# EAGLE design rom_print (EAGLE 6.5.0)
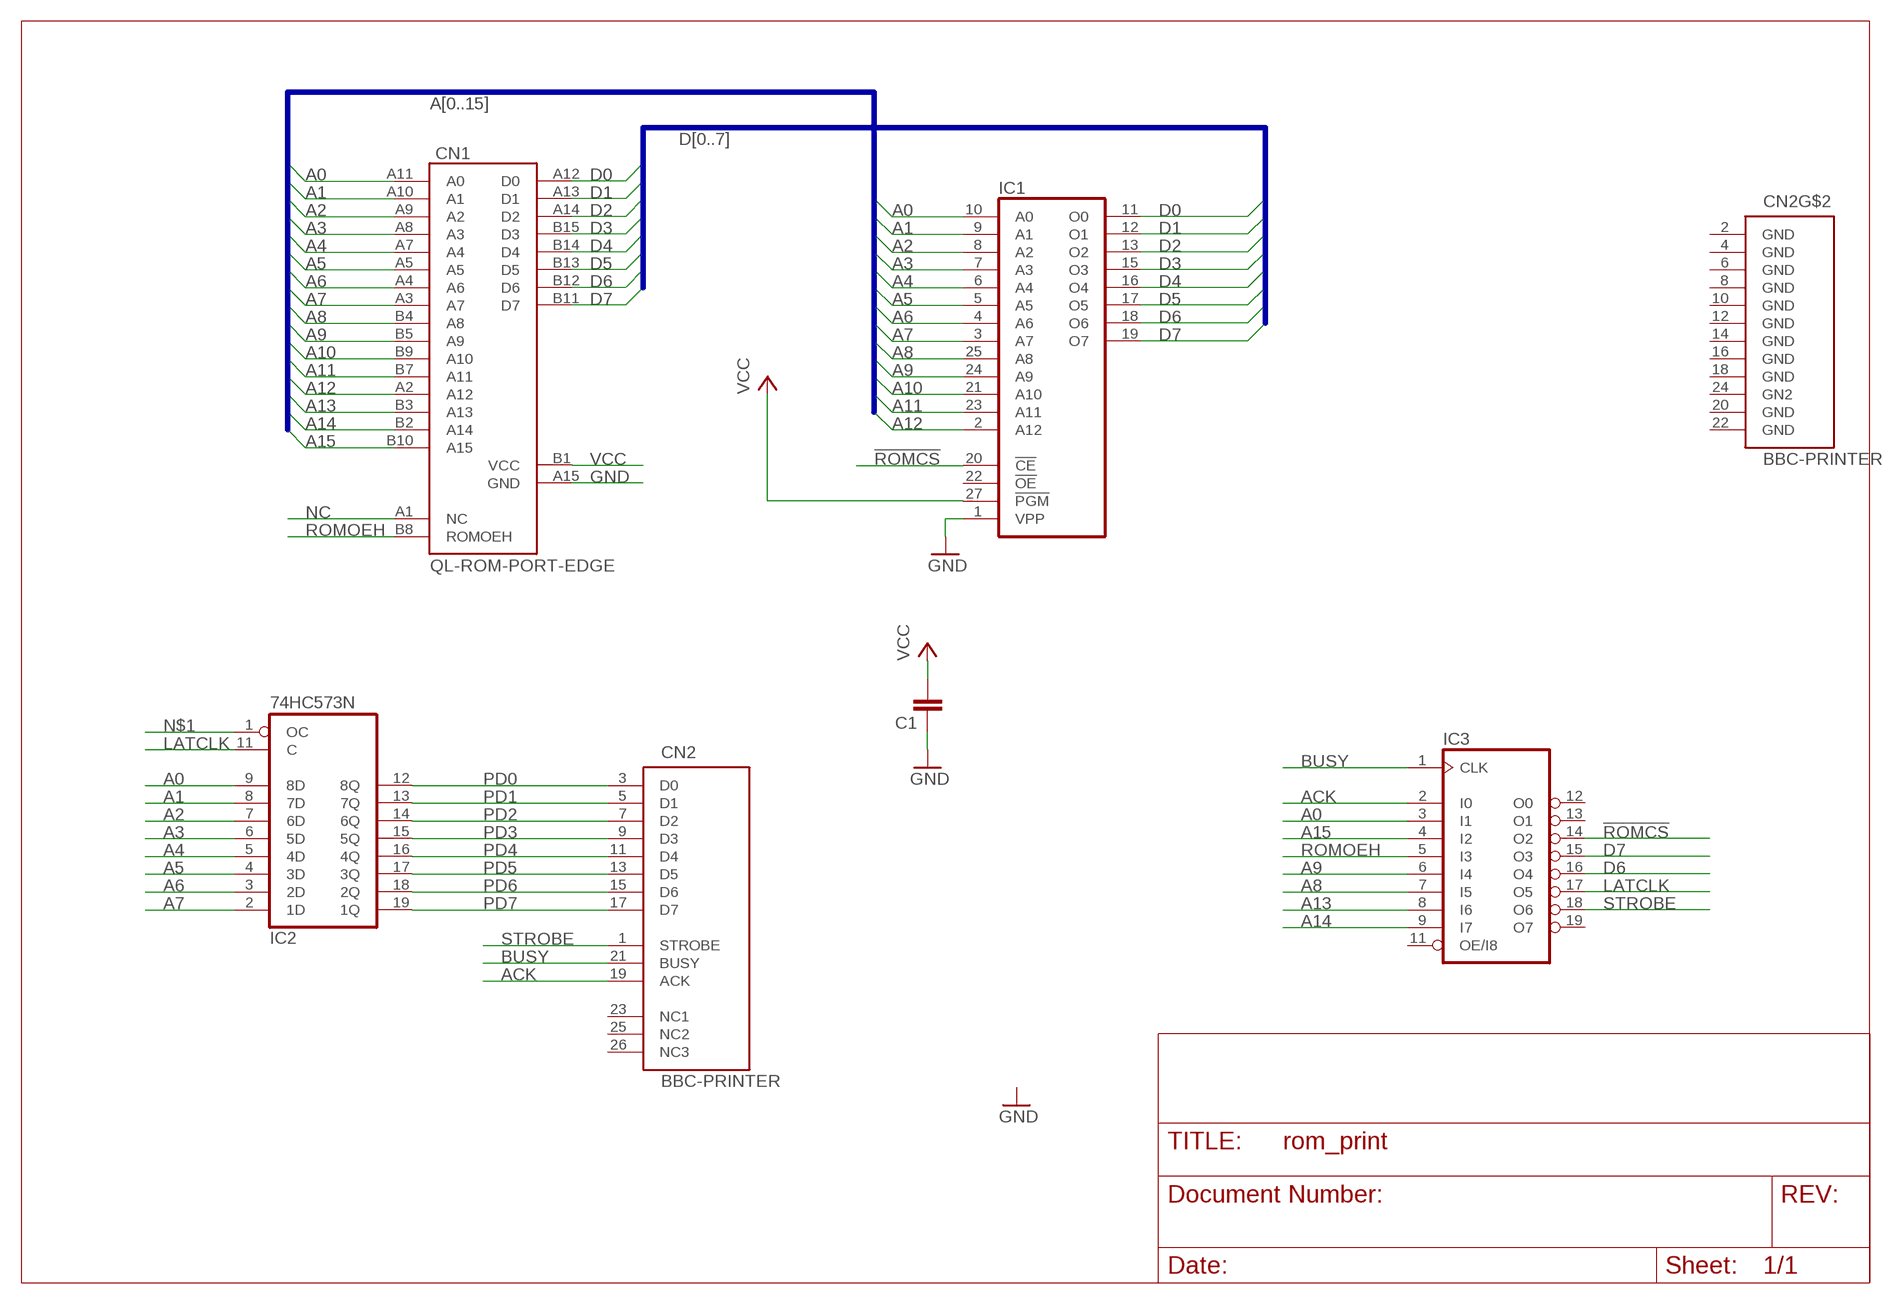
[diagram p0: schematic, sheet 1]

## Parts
C1  C-EU025_050-025X075  [C025_050-025X075]
CN1  QL-ROM-PORT-EDGE  [QL-ROM-WDGE]
CN2  BBC-PRINTER  [2X13]
IC1  2764  [DIL28]
IC2  74HC573N  [DIL20]
IC3  16V8  [DIL20]

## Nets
!ROMCS: IC1.20(!CE) IC3.14(O2)
A0: CN1.A11(A0) IC1.10(A0) IC2.9(8D) IC3.3(I1)
A1: CN1.A10(A1) IC1.9(A1) IC2.8(7D)
A2: CN1.A9(A2) IC1.8(A2) IC2.7(6D)
A3: CN1.A8(A3) IC1.7(A3) IC2.6(5D)
A4: CN1.A7(A4) IC1.6(A4) IC2.5(4D)
A5: CN1.A5 IC1.5(A5) IC2.4(3D)
A6: CN1.A4(A6) IC1.4(A6) IC2.3(2D)
A7: CN1.A3(A7) IC1.3(A7) IC2.2(1D)
A8: CN1.B4(A8) IC1.25(A8) IC3.7(I5)
A9: CN1.B5(A9) IC1.24(A9) IC3.6(I4)
A10: CN1.B9(A10) IC1.21(A10)
A11: CN1.B7(A11) IC1.23(A11)
A12: CN1.A2(A12) IC1.2(A12)
A13: CN1.B3(A13) IC3.8(I6)
A14: CN1.B2(A14) IC3.9(I7)
A15: CN1.B10(A15) IC3.4(I2)
ACK: CN2.19(ACK) IC3.2(I0)
BUSY: CN2.21(BUSY) IC3.1(CLK)
D0: CN1.A12(D0) IC1.11(O0)
D1: CN1.A13(D1) IC1.12(O1)
D2: CN1.A14(D2) IC1.13(O2)
D3: CN1.B15(D3) IC1.15(O3)
D4: CN1.B14(D4) IC1.16(O4)
D5: CN1.B13(D5) IC1.17(O5)
D6: CN1.B12(D6) IC1.18(O6) IC3.16(O4)
D7: CN1.B11(D7) IC1.19(O7) IC3.15(O3)
GND: C1.1 CN1.A15(GND) IC1.1(VPP)
LATCLK: IC2.11(C) IC3.17(O5)
N$1: IC2.1(OC)
NC: CN1.A1(NC)
PD0: CN2.3(D0) IC2.12(8Q)
PD1: CN2.5(D1) IC2.13(7Q)
PD2: CN2.7(D2) IC2.14(6Q)
PD3: CN2.9(D3) IC2.15(5Q)
PD4: CN2.11(D4) IC2.16(4Q)
PD5: CN2.13(D5) IC2.17(3Q)
PD6: CN2.15(D6) IC2.18(2Q)
PD7: CN2.17(D7) IC2.19(1Q)
ROMOEH: CN1.B8(ROMOEH) IC3.5(I3)
STROBE: CN2.1(STROBE) IC3.18(O6)
VCC: C1.2 CN1.B1(VCC) IC1.27(!PGM)
Unconnected: CN2.23(NC1) CN2.25(NC2) CN2.26(NC3) IC1.22(!OE) IC3.11(OE/I8) IC3.12(O0) IC3.13(O1) IC3.19(O7)

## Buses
A[0..15]
D[0..7]

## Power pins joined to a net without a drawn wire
GN2: CN2.24(GN2)
GND: CN2.2(GND) CN2.4(GND) CN2.6(GND) CN2.8(GND) CN2.10(GND) CN2.12(GND) CN2.14(GND) CN2.16(GND) CN2.18(GND) CN2.20(GND) CN2.22(GND) IC1.14(GND) IC2.10(GND) IC3.10(GND)
VCC: IC1.28(VCC) IC2.20(VCC) IC3.20(VCC)

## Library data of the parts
C1 = rcl:C-EU: CAPACITOR, European symbol
CN1 = Con-Sinclair:QL-ROM-PORT-EDGE: Sinclair QL romsocket ege connector
CN2 = Con-Acorn:BBC-PRINTER: BBC Micro printer port
IC1 = memory:2764: MEMORY
IC2 = 74xx-eu:74*573: 8-bit D latch BUS DRIVER
IC3 = pal:16V8: PAL; MPN: GAL16V8D-7LPN; OC_FARNELL: 9699740; OC_NEWARK: 97K0449

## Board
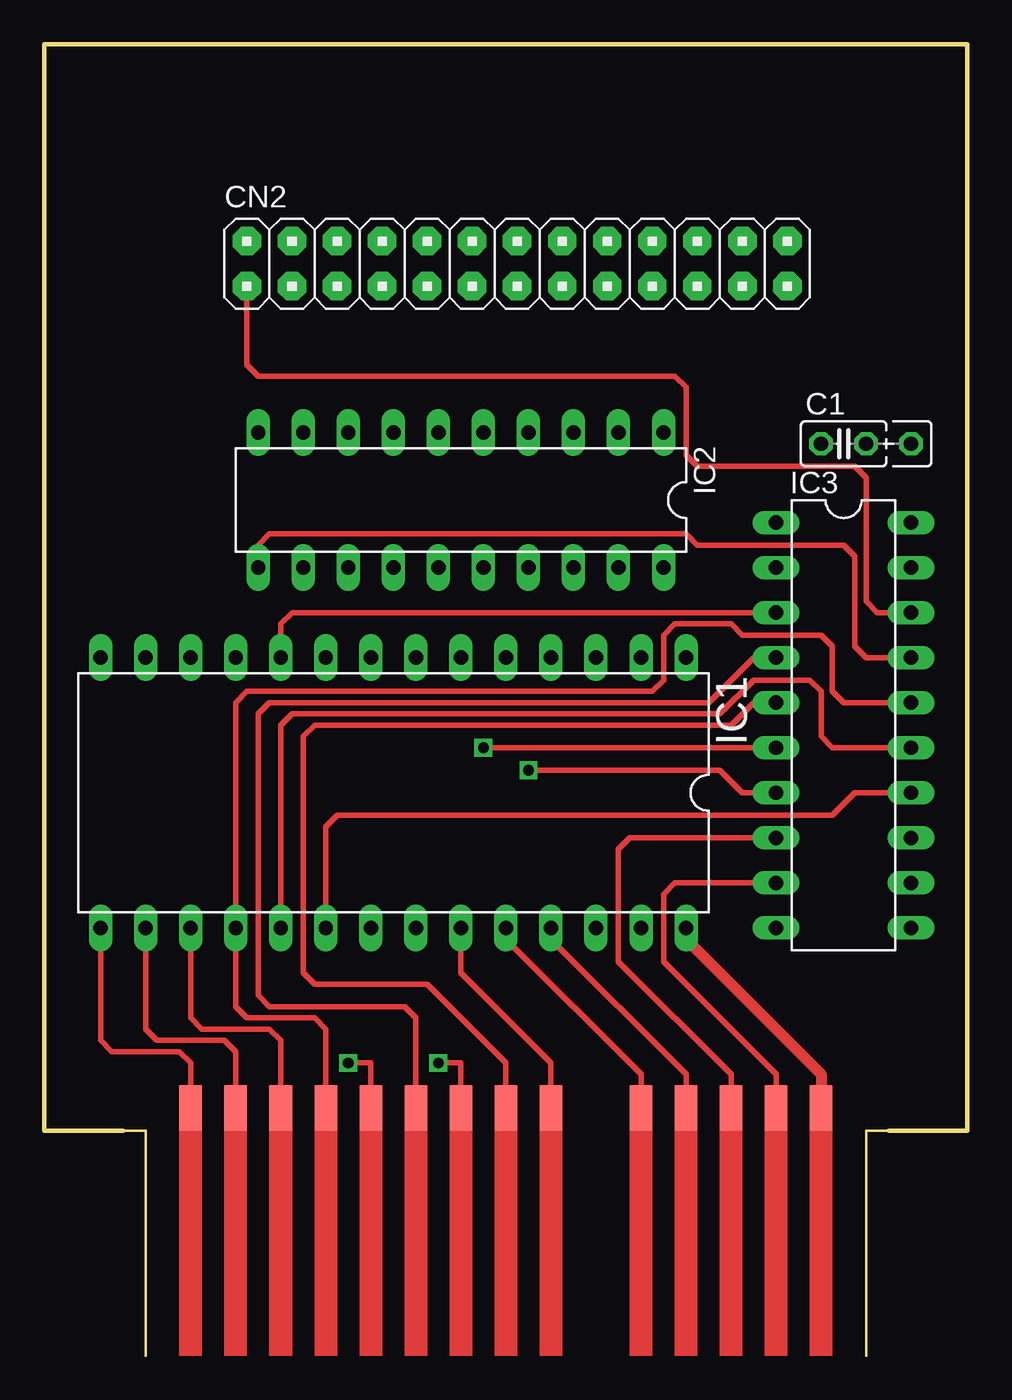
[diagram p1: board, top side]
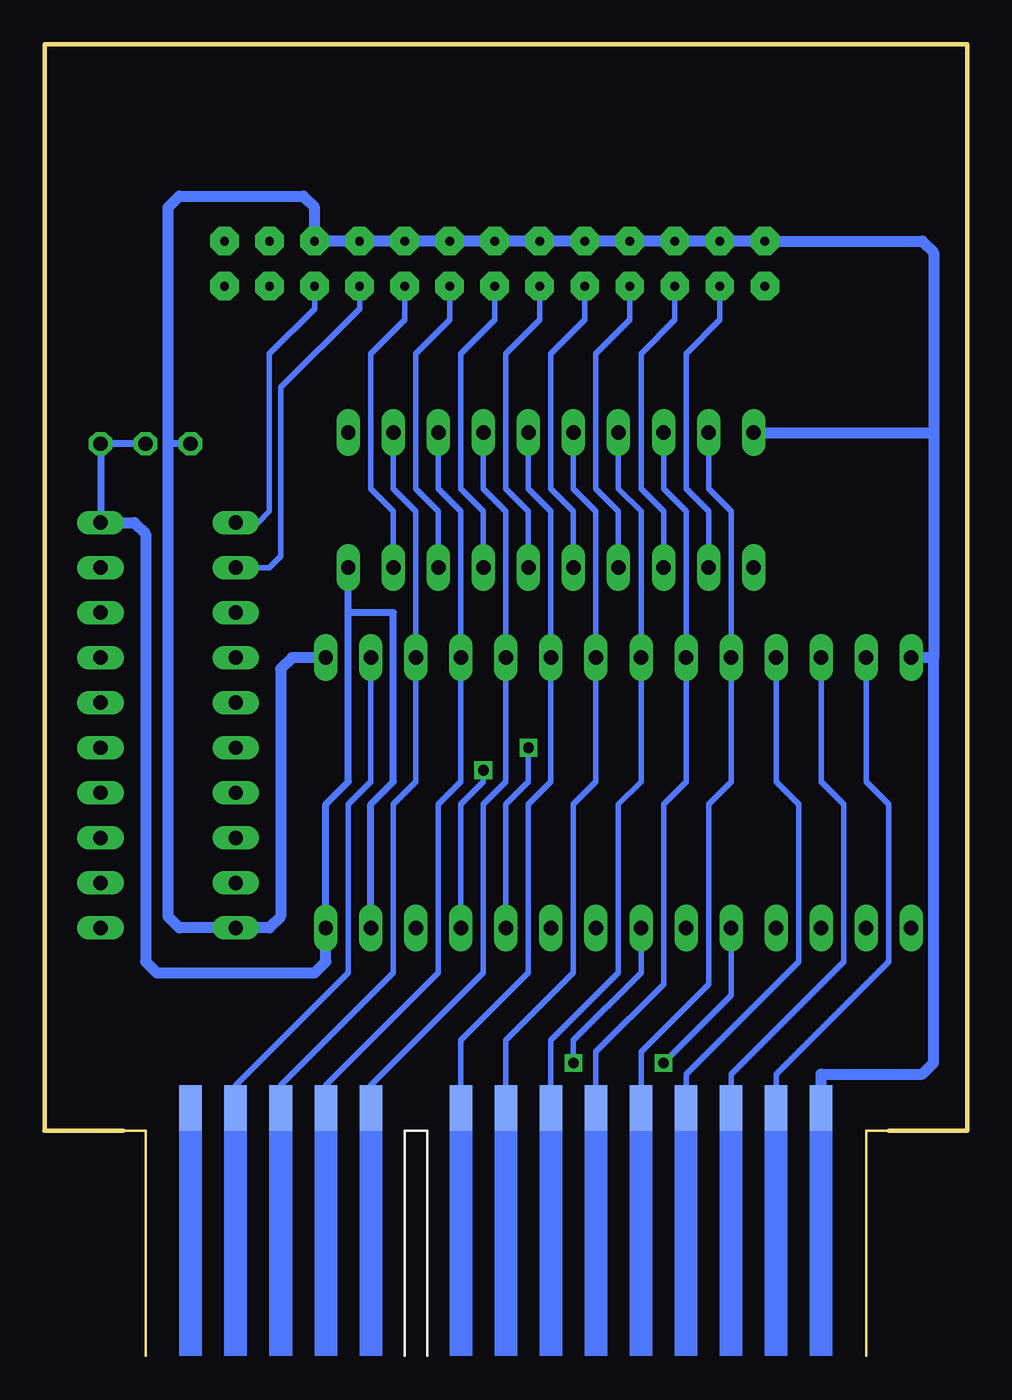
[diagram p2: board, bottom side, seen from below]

Size 52.07 x 73.97 mm. Coordinates in mm from the lower left corner, seen from the top.
Outline: 52.05,12.7 52.05,73.97 0,73.97 0,12.7 4.45,12.7
Outline: 47.62,12.7 52.05,12.7
Outline: 52.05,12.7 52.07,12.7
Copper layers (1*16): Top 0.035mm / dielectric 1.5mm / Bottom 0.035mm
Design rules "default": minimum track width 10mil, minimum drill 24mil, track to track 8mil, track to pad 8mil, pad to pad 8mil, via to via 8mil, smd to smd 8mil, copper to edge 40mil, drill to drill 8mil, minimum pad ring 10mil, minimum via ring 8mil, stop-mask expansion 4mil, vias tented up to drill 0mil, thermal gap 10mil

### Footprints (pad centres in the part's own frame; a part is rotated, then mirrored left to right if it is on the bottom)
C025_050-025X075 = drill 0.813 octagon: 1 -1.27,0; 2 1.27,0; 3 3.81,0
QL-ROM-WDGE = smd 1.27 x 2.54 bottom: A1 39.37,15.24; A2 36.83,15.24; A3 34.29,15.24; A4 31.75,15.24; A5 29.21,15.24; A7 24.13,15.24; A8 21.59,15.24; A9 19.05,15.24; A10 16.51,15.24; A11 13.97,15.24; A12 11.43,15.24; A13 8.89,15.24; A14 6.35,15.24; A15 3.81,15.24 | smd 1.27 x 2.54: B1 39.37,15.24; B2 36.83,15.24; B3 34.29,15.24; B4 31.75,15.24; B5 29.21,15.24; B7 24.13,15.24; B8 21.59,15.24; B9 19.05,15.24; B10 16.51,15.24; B11 13.97,15.24; B12 11.43,15.24; B13 8.89,15.24; B14 6.35,15.24; B15 3.81,15.24
2X13 = drill 0.5 pad 1.6 octagon: 1 -15.24,-1.27; 2 -15.24,1.27; 3 -12.7,-1.27; 4 -12.7,1.27; 5 -10.16,-1.27; 6 -10.16,1.27; 7 -7.62,-1.27; 8 -7.62,1.27; 9 -5.08,-1.27; 10 -5.08,1.27; 11 -2.54,-1.27; 12 -2.54,1.27; 13 0,-1.27; 14 0,1.27; 15 2.54,-1.27; 16 2.54,1.27; 17 5.08,-1.27; 18 5.08,1.27; 19 7.62,-1.27; 20 7.62,1.27; 21 10.16,-1.27; 22 10.16,1.27; 23 12.7,-1.27; 24 12.7,1.27; 25 15.24,-1.27; 26 15.24,1.27
DIL28 = drill 0.813 long: 1 -16.51,-7.62; 2 -13.97,-7.62; 3 -11.43,-7.62; 4 -8.89,-7.62; 5 -6.35,-7.62; 6 -3.81,-7.62; 7 -1.27,-7.62; 8 1.27,-7.62; 9 3.81,-7.62; 10 6.35,-7.62; 11 8.89,-7.62; 12 11.43,-7.62; 13 13.97,-7.62; 14 16.51,-7.62; 15 16.51,7.62; 16 13.97,7.62; 17 11.43,7.62; 18 8.89,7.62; 19 6.35,7.62; 20 3.81,7.62; 21 1.27,7.62; 22 -1.27,7.62; 23 -3.81,7.62; 24 -6.35,7.62; 25 -8.89,7.62; 26 -11.43,7.62; 27 -13.97,7.62; 28 -16.51,7.62
DIL20 = drill 0.813 long: 1 -11.43,-3.81; 2 -8.89,-3.81; 3 -6.35,-3.81; 4 -3.81,-3.81; 5 -1.27,-3.81; 6 1.27,-3.81; 7 3.81,-3.81; 8 6.35,-3.81; 9 8.89,-3.81; 10 11.43,-3.81; 11 11.43,3.81; 12 8.89,3.81; 13 6.35,3.81; 14 3.81,3.81; 15 1.27,3.81; 16 -1.27,3.81; 17 -3.81,3.81; 18 -6.35,3.81; 19 -8.89,3.81; 20 -11.43,3.81

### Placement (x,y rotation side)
C1  45.09,51.43 0 top
CN1  4.45,-1.27 0 top
CN2  26.67,61.59 0 top
IC1  19.68,31.75 180 top
IC2  23.5,48.26 180 top
IC3  45.09,35.56 270 top

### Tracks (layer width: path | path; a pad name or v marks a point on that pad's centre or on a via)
!ROMCS
  Top 0.305: IC1.20 15.88,29.84 16.51,30.48 44.45,30.48 45.72,31.75 IC3.14
A0
  Top 0.305: IC3.3 13.97,41.91 13.34,41.27 IC1.10
  Bottom 0.305: CN1.A11 18.41,17.14 14.61,20.96 14.61,31.11 13.34,32.38 IC1.10 13.34,47.62 14.61,48.89 IC2.9
A1
  Bottom 0.305: CN1.A10 20.95,17.14 17.14,20.96 17.14,31.11 15.88,32.38 IC1.9 15.88,47.62 17.14,48.89 IC2.8
A2
  Bottom 0.305: CN1.A9 23.5,17.78 19.68,21.59 19.68,31.11 18.41,32.38 IC1.8 18.41,47.62 19.68,48.89 IC2.7
A3
  Bottom 0.305: CN1.A8 26.04,17.78 22.23,21.59 22.23,31.11 20.95,32.38 IC1.7 20.95,47.62 22.23,48.89 IC2.6
A4
  Bottom 0.305: CN1.A7 28.57,17.78 24.77,21.59 24.77,31.11 23.5,32.38 IC1.6 23.5,47.62 24.77,48.89 IC2.5
A5
  Bottom 0.305: CN1.A5 33.66,15.24 27.3,21.59 27.3,31.11 26.04,32.38 IC1.5 26.04,47.62 27.3,48.89 IC2.4
A6
  Bottom 0.305: 36.2,13.34 CN1.A4 36.2,15.24 29.84,21.59 29.84,31.11 28.57,32.38 IC1.4 28.57,47.62 29.84,48.89 IC2.3
A7
  Bottom 0.305: CN1.A3 38.73,15.24 32.38,21.59 32.38,31.11 31.11,32.38 IC1.3 31.11,47.62 32.38,48.89 IC2.2
A8  (via drill 0.6)
  Top 0.305: CN1.B4 36.2,15.88 28.57,23.5 IC1.25 | v27.3,33.02 38.1,33.02 39.37,31.75 IC3.7
  Bottom 0.305: IC1.25 28.57,31.11 27.3,32.38 v27.3,33.02
A9  (via drill 0.6)
  Top 0.305: CN1.B5 33.66,15.88 26.04,23.5 IC1.24 | v24.77,34.29 IC3.6
  Bottom 0.305: IC1.24 26.04,31.11 24.77,32.38 v24.77,34.29
A10  (via drill 0.6)
  Top 0.305: v22.23,16.51 23.5,16.51 CN1.B9
  Bottom 0.305: IC1.21 18.41,21.59 22.23,17.78 v22.23,16.51
A11
  Top 0.305: CN1.B7 28.57,16.51 23.5,21.59 IC1.23
A12
  Bottom 0.305: IC1.2 33.66,32.38 34.92,31.11 34.92,21.59 41.27,15.24 CN1.A2
A13
  Top 0.305: CN1.B3 38.73,15.88 32.38,22.23 32.38,28.57 33.02,29.21 IC3.8
A14
  Top 0.305: CN1.B2 41.27,15.88 34.92,22.23 34.92,26.04 35.56,26.67 IC3.9
A15
  Top 0.305: CN1.B10 20.95,19.05 20.32,19.68 12.7,19.68 12.06,20.32 12.06,36.2 12.7,36.83 37.47,36.83 40.01,39.37 IC3.4
ACK
  Bottom 0.305: IC3.2 39.37,44.45 38.73,45.08 38.73,54.61 34.29,59.05 CN2.19
BUSY
  Bottom 0.305: IC3.1 40.01,46.99 39.37,47.62 39.37,56.51 36.83,59.05 CN2.21
D0
  Bottom 0.305: CN1.A12 15.88,15.88 9.53,22.23 9.53,31.11 10.79,32.38 IC1.11
D1
  Bottom 0.305: IC1.12 8.26,32.38 6.99,31.11 6.99,22.23 13.34,15.88 CN1.A13
D2
  Bottom 0.305: CN1.A14 10.79,15.88 4.45,22.23 4.45,31.11 5.71,32.38 IC1.13
D3
  Top 0.305: CN1.B15 8.26,16.51 7.62,17.14 3.81,17.14 3.17,17.78 IC1.15
D4
  Top 0.305: CN1.B14 10.79,17.14 10.16,17.78 6.35,17.78 5.71,18.41 IC1.16
D5
  Top 0.305: CN1.B13 13.34,17.78 12.7,18.41 8.89,18.41 8.26,19.05 IC1.17
D6
  Top 0.305: CN1.B12 15.88,18.41 15.24,19.05 11.43,19.05 10.79,19.68 IC1.18 10.79,36.83 11.43,37.46 34.29,37.46 34.92,38.1 34.92,40.64 35.56,41.27 38.73,41.27 39.37,40.64 43.81,40.64 44.45,40 44.45,37.46 45.09,36.83 IC3.16
D7  (via drill 0.6)
  Top 0.305: v17.14,16.51 18.41,16.51 CN1.B11 | IC3.15 44.45,34.29 43.81,34.92 43.81,37.46 43.18,38.1 40.01,38.1 38.1,36.2 13.97,36.2 13.34,35.56 IC1.19
  Bottom 0.305: IC1.19 13.34,20.32 v17.14,16.51
GND
  Bottom 0.406: C1.1 45.09,51.43
  Bottom 0.61: CN1.A15 8.26,15.88 2.54,15.88 1.91,16.51 1.91,39.37 | 1.91,39.37 IC1.14 | IC2.10 1.91,52.07 | 1.91,52.07 1.91,39.37 | 1.91,52.07 1.91,62.23 2.54,62.87 CN2.2 CN2.4 CN2.6 CN2.8 CN2.10 CN2.12 CN2.14 CN2.16 CN2.18 CN2.20 CN2.22 36.83,64.77 37.47,65.41 44.45,65.41 45.09,64.77 45.09,51.43 45.09,24.77 44.45,24.13 IC3.10 39.37,24.13 38.73,24.77 38.73,38.73 38.1,39.37 IC1.1
LATCLK
  Top 0.305: IC3.17 46.35,39.37 45.72,40 45.72,45.08 45.09,45.72 36.83,45.72 36.2,46.35 12.7,46.35 12.06,45.72 IC2.11
PD0
  Bottom 0.305: IC2.12 14.61,47.62 15.88,48.89 15.88,56.51 13.97,58.42 CN2.3
PD1
  Bottom 0.305: IC2.13 17.14,47.62 18.41,48.89 18.41,56.51 16.51,58.42 CN2.5
PD2
  Bottom 0.305: IC2.14 19.68,47.62 20.95,48.89 20.95,56.51 19.05,58.42 CN2.7
PD3
  Bottom 0.305: IC2.15 22.23,47.62 23.5,48.89 23.5,56.51 21.59,58.42 CN2.9
PD4
  Bottom 0.305: IC2.16 24.77,47.62 26.04,48.89 26.04,56.51 24.13,58.42 CN2.11
PD5
  Bottom 0.305: IC2.17 27.3,47.62 28.57,48.89 28.57,56.51 26.67,58.42 CN2.13
PD6
  Bottom 0.305: IC2.18 29.84,47.62 31.11,48.89 31.11,56.51 29.21,58.42 CN2.15
PD7
  Bottom 0.305: IC2.19 32.38,47.62 33.66,48.89 33.66,56.51 31.75,58.42 CN2.17
ROMOEH
  Top 0.305: CN1.B8 26.04,16.51 21.59,20.96 15.24,20.96 14.61,21.59 14.61,34.92 15.24,35.56 38.73,35.56 40.01,36.83 IC3.5
STROBE
  Top 0.305: IC3.18 46.99,41.91 46.35,42.54 46.35,49.53 45.72,50.16 36.83,50.16 36.2,50.8 36.2,54.61 35.56,55.24 12.06,55.24 11.43,55.88 CN2.1
VCC
  Top 0.61: IC1.28 36.2,23.5 43.81,15.88 CN1.B1
  Bottom 0.406: IC1.28 36.2,31.11 34.92,32.38 34.92,41.91 | 34.92,41.91 IC2.20 | IC1.27 33.66,31.11 32.38,32.38 32.38,41.91 34.92,41.91 | C1.2 48.9,51.43 IC3.20
  Bottom 0.61: IC3.20 46.99,46.99 46.35,46.35 46.35,22.23 45.72,21.59 36.83,21.59 36.2,22.23 IC1.28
